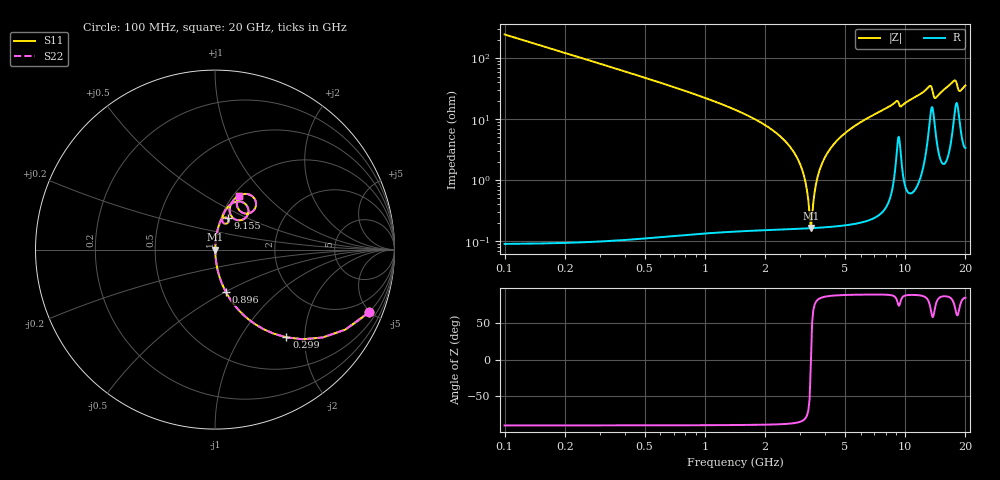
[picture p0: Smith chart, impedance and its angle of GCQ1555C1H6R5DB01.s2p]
!Murata Part Number: GCQ1555C1H6R5DB01
!These Parameters are Measured in Series Mode Connection
!Data Generated on Mar 13, 2026
!  o--ll--o
!Port1  Port2
!  o------o
!Operation Temp=25[degC], DC Bias Voltage=0[V]
!Freq. Start=100[MHz] Stop=20[GHz] 401[Steps]
# Hz S RI R 50
!Freq.(Hz) S11(Real) S11(Imag) S21(Real) S21(Imag) S12(Real) S12(Imag) S22(Real) S22(Imag)
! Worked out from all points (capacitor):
!   401 points, 100 MHz to 20 GHz, reference 50 ohm
!   read as one part in series: C = 6.5 pF near 199.5 MHz
!   lowest |Z| = 163 mohm at 3.384 GHz (marker M1)
!   series resonance near 3.387 GHz, so ESL is about 340 pH
!   S11 on the Smith chart (normalised r, x): 100 MHz: 1.00, -4.89; 299 MHz: 1.00, -1.62; 896 MHz: 1.00, -0.51; 9.155 GHz: 1.08, +0.39; 20 GHz: 1.07, +0.71
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1e8  0.8567 -0.3502  0.1433 0.3502  0.1433 0.3502  0.8567 -0.3502
2.99e8  0.3977 -0.4888  0.6023 0.4888  0.6023 0.4888  0.3977 -0.4888
5.4775e8  0.1598 -0.3651  0.8402 0.3651  0.8402 0.3651  0.1598 -0.3651
8.96e8  0.0617 -0.238  0.9383 0.238  0.9383 0.238  0.0617 -0.238
2.73675e9  0.00253 -0.031  0.9975 0.031  0.9975 0.031  0.00253 -0.031
3.085e9  0.00178 -0.0135  0.9982 0.0135  0.9982 0.0135  0.00178 -0.0135
3.3835e9  0.00162 -0.000137  0.9984 0.000137  0.9984 0.000137  0.00162 -0.000137
3.43325e9  0.00163 0.00198  0.9984 -0.00198  0.9984 -0.00198  0.00163 0.00198
3.5825e9  0.00171 0.00815  0.9983 -0.00815  0.9983 -0.00815  0.00171 0.00815
3.73175e9  0.00185 0.0141  0.9981 -0.0141  0.9981 -0.0141  0.00185 0.0141
4.22925e9  0.00276 0.0325  0.9972 -0.0325  0.9972 -0.0325  0.00276 0.0325
5.1745e9  0.00589 0.0636  0.9941 -0.0636  0.9941 -0.0636  0.00589 0.0636
6.7665e9  0.0145 0.1099  0.9855 -0.1099  0.9855 -0.1099  0.0145 0.1099
9.1545e9  0.0697 0.1746  0.9303 -0.1746  0.9303 -0.1746  0.0697 0.1746
9.50275e9  0.0497 0.1467  0.9503 -0.1467  0.9503 -0.1467  0.0497 0.1467
1.005e10  0.0401 0.1767  0.9599 -0.1767  0.9599 -0.1767  0.0401 0.1767
1.338325e10  0.1774 0.2441  0.8226 -0.2441  0.8226 -0.2441  0.1774 0.2441
1.407975e10  0.1048 0.1728  0.8952 -0.1728  0.8952 -0.1728  0.1048 0.1728
1.67165e10  0.1387 0.3037  0.8613 -0.3037  0.8613 -0.3037  0.1387 0.3037
1.77115e10  0.2201 0.2835  0.7799 -0.2835  0.7799 -0.2835  0.2201 0.2835
1.865675e10  0.1431 0.2117  0.8569 -0.2117  0.8569 -0.2117  0.1431 0.2117
2e10  0.1349 0.2977  0.8651 -0.2977  0.8651 -0.2977  0.1349 0.2977
